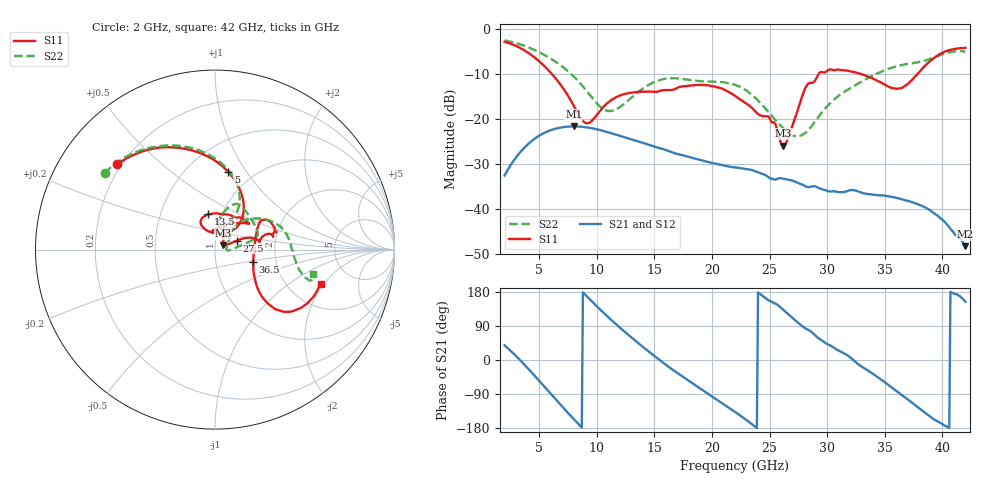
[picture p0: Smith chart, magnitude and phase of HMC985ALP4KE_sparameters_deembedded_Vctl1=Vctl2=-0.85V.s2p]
!s2p File: Measurements: S11, S21, S12, S22
# GHz S dB R 50.0
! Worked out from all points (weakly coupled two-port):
!   401 points, 2 GHz to 42 GHz, reference 50 ohm
!   highest |S21| = -21.66 dB at 8 GHz (marker M1); lowest = -48.3 dB at 42 GHz (marker M2)
!   lowest |S11| = -25.9 dB at 26.2 GHz (marker M3), VSWR 1.11, Z = 54.6 + j2.71 ohm
!   |S11| at or under -10 dB: 6.113 GHz to 29.26 GHz (23.14 GHz wide, 131 % of centre); 32.96 GHz to 37.84 GHz (4.88 GHz wide, 13.8 % of centre)
!   |S22| runs from -23.9 to -2.5 dB; largest |S21 - S12| = 0.00013
!   S11 on the Smith chart (normalised r, x): 2 GHz: 0.18, +0.36; 5 GHz: 0.77, +0.83; 13.5 GHz: 0.86, +0.35; 27.5 GHz: 1.27, +0.13; 36.5 GHz: 1.52, -0.21; 42 GHz: 2.98, -1.87
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2  -2.83 138.8  -32.59 38.7  -32.59 38.7  -2.52 145.3
3.4  -4.26 111.7  -27.29 -2.2  -27.29 -2.2  -3.43 122.7
5  -7.14 80.4  -23.73 -54.9  -23.73 -54.9  -5.13 98.0
6.3  -10.56 57.4  -22.25 -99.3  -22.26 -99.3  -7.05 79.8
8  -17.02 48.1  -21.66 -155.9  -21.66 -155.9  -10.53 62.6
8.7  -20.13 63.8  -21.74 -178.3  -21.75 -178.3  -12.47 59.6
9.4  -20.78 93.3  -21.99 159.9  -21.99 159.9  -14.66 60.1
11  -16.30 119.0  -22.98 112.9  -22.98 112.9  -18.23 76.3
13.5  -13.99 100.5  -24.93 47.1  -24.93 47.1  -14.20 79.4
15.4  -13.83 74.6  -26.44 1.5  -26.45 1.5  -11.39 68.3
18.9  -12.44 38.5  -29.08 -73.7  -29.09 -73.7  -11.55 41.0
22  -14.83 54.6  -30.78 -137.0  -30.79 -137.0  -12.40 16.5
24.9  -19.45 92.7  -32.94 157.7  -32.95 157.7  -18.44 5.9
26.2  -25.91 29.3  -33.30 131.8  -33.30 131.8  -22.16 -3.1
27.5  -17.58 22.1  -34.28 97.6  -34.25 97.5  -23.83 4.5
28.7  -11.94 10.0  -35.03 72.4  -35.00 72.3  -21.43 29.4
31  -9.03 20.8  -36.30 24.7  -36.30 24.6  -14.81 49.6
33.3  -10.31 32.1  -36.62 -23.1  -36.63 -23.1  -11.26 39.1
35.4  -12.87 10.9  -37.28 -67.8  -37.26 -67.6  -8.78 24.4
36.5  -13.08 -17.6  -37.91 -92.8  -37.90 -92.6  -7.97 15.6
39.6  -5.85 -42.6  -41.58 -162.2  -41.64 -162.9  -6.00 -15.4
42  -4.16 -18.2  -48.33 153.6  -48.25 153.4  -4.99 -13.8
